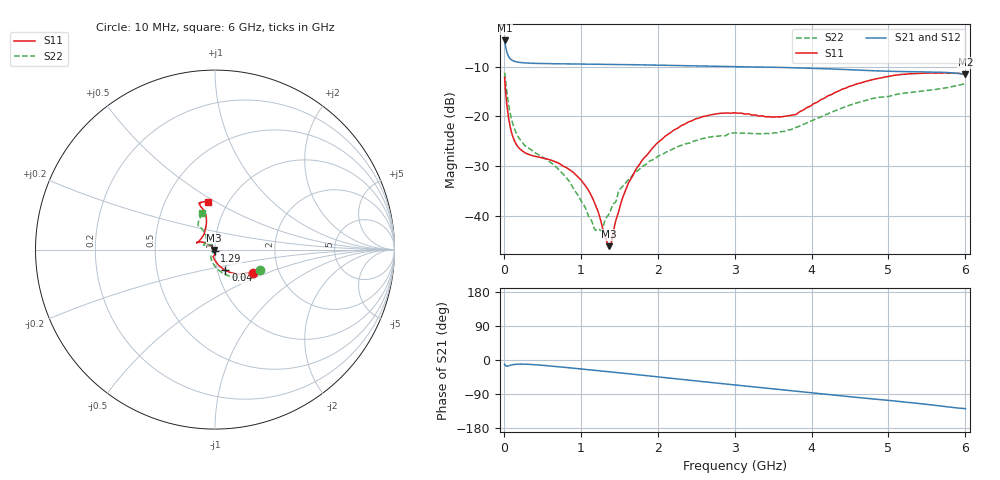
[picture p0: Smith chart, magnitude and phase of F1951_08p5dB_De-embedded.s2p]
! Integrated Device Technology
! Corporate Headquarters
! 6024 Silver Creek Valley Road
! San Jose, CA 95138  USA
! Phone:  1-408-284-8200
! Toll Free:  1-800-223-1366
! Webpage:  http://www.idt.com/
! Timing and RF Division
! 515 Groton Road, Suite 102
! Westford, MA 01886-6024
! Device:  F1951
! Description: 6-bit 0.5 dB Digital Step Attenuator
! Frequency:  100.0 -  4000.00 MHz
! Package:  4x4 mm Thin QFN Plastic Package: 24 pin
! Ports:  2 RF, 6 DC
!  Pin  1  = NC
!  Pin  2  = RF1  =  Port 1
!  Pin  3  = GND
!  Pin  4  = NC
!  Pin  5  = Serial Data Out (SDO)
!  Pin  6  = NC
!  Pin  7  = Reset Bar ( RSTb)
!  Pin  8  = Clock (CLK)
!  Pin  9  = Chip Select Bar (CSb)
!  Pin 10  = NC
!  Pin 11  = Serial Data In (SDI)
!  Pin 12  = NC
!  Pin 13  = NC
!  Pin 14  = VDD
!  Pin 15  = NC
!  Pin 16  = GND
!  Pin 17  = RF2  =  Port 2
!  Pin 18  = NC
!  Pin 19  = GND
!  Pin 20  = GND
!  Pin 21  = GND
!  Pin 22  = GND
!  Pin 23  = GND
!  Pin 24  = GND
! State:  17
! Atten State:  8.5 dB
! Voltage:  +3.30 Volts
! Current:  0.488 mA
! Data:  The device was measured on a F195X evaluation board which has
!  individual transmission lines to the RF pins.  Data was collected
!  de-embedded using a Automatic Fixture Removal [AFR] (Keysight Technologies).
!  The reference plane is the edge of the package pin.
! Misc:  Lot Code  1225BCA
!  Action Tracker AT0399
! Date Measured:  2018-09-13
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# GHz S dB R 50
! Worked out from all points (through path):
!   600 points, 10 MHz to 6 GHz, reference 50 ohm
!   highest |S21| = -4.66 dB at 10 MHz (marker M1); lowest = -11.5 dB at 6 GHz (marker M2)
!   group delay of S21, straight-line fit = 57 ps
!   lowest |S11| = -46.2 dB at 1.37 GHz (marker M3), VSWR 1.01, Z = 49.5 - j0.162 ohm
!   |S11| at or under -10 dB: start of sweep to end of sweep
!   |S22| runs from -43.0 to -11.2 dB; largest |S21 - S12| = 0.00052
!   S11 on the Smith chart (normalised r, x): 10 MHz: 1.47, -0.40; 40 MHz: 1.09, -0.26; 1.29 GHz: 0.99, -0.01; 6 GHz: 0.81, +0.46
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0.01  -12.14 -31.4  -4.66 -11.0  -4.66 -11.0  -11.16 -23.9
0.04  -17.77 -63.2  -7.02 -16.3  -7.02 -16.4  -15.17 -59.5
0.07  -21.05 -76.9  -8.10 -14.7  -8.10 -14.8  -18.36 -78.2
0.1  -23.23 -85.1  -8.58 -13.0  -8.58 -13.0  -20.58 -89.6
0.2  -26.41 -99.1  -9.08 -10.9  -9.08 -10.9  -24.42 -109.7
0.76  -29.92 -96.2  -9.38 -18.7  -9.38 -18.8  -31.47 -123.7
1.01  -32.96 -89.8  -9.44 -23.7  -9.44 -23.7  -37.21 -126.9
1.19  -37.85 -94.7  -9.46 -27.3  -9.46 -27.3  -43.00 -163.4
1.29  -42.97 -111.6  -9.47 -29.4  -9.48 -29.4  -42.31 154.2
1.37  -46.19 -160.5  -9.49 -31.1  -9.49 -31.1  -39.60 137.9
1.4  -45.26 175.3  -9.50 -31.7  -9.50 -31.7  -38.45 132.2
1.51  -38.21 142.6  -9.52 -33.9  -9.53 -33.9  -34.67 126.2
1.62  -33.44 137.5  -9.54 -36.3  -9.54 -36.3  -32.76 123.0
1.8  -28.79 137.7  -9.58 -40.2  -9.58 -40.2  -30.10 125.9
2.01  -25.15 142.8  -9.64 -44.7  -9.64 -44.7  -27.96 133.0
2.49  -20.50 153.3  -9.79 -55.0  -9.79 -55.0  -24.89 149.1
3.01  -19.26 159.4  -9.95 -65.9  -9.96 -65.8  -23.30 155.7
3.6  -20.10 137.5  -10.10 -78.3  -10.10 -78.3  -23.07 136.5
4.01  -17.62 113.1  -10.27 -87.0  -10.27 -87.0  -20.85 123.1
4.5  -13.89 105.0  -10.58 -97.0  -10.58 -97.0  -17.71 122.0
5.01  -11.90 108.6  -10.89 -106.8  -10.89 -106.8  -15.93 124.5
6  -11.49 98.1  -11.46 -128.4  -11.46 -128.4  -13.38 109.3
